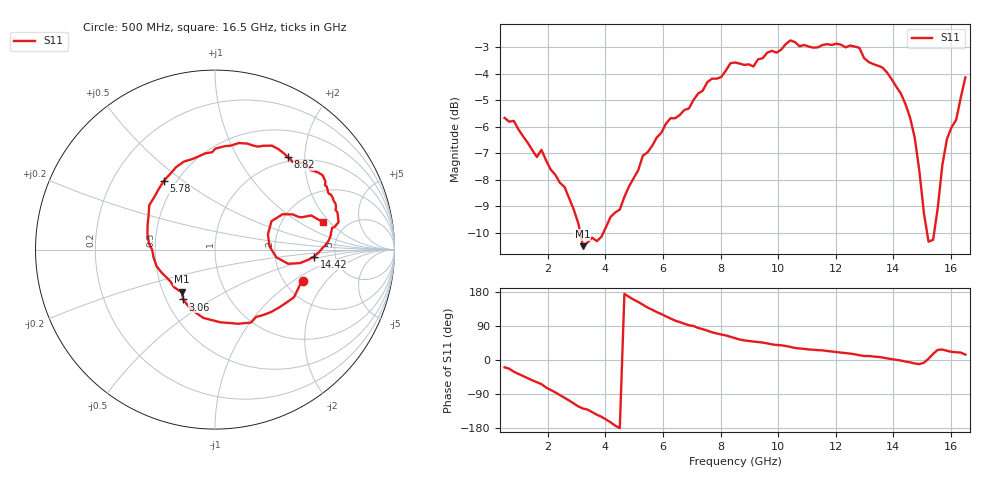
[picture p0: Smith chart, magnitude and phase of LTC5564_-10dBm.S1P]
! LTC5564 S11 -10 dBm source power.
! Reference plane is 1.1 mm from edge of QFN package.
! Measured 11-Jan 2013
# GHZ S DB R 50
!GHz	dB_S11	angS11
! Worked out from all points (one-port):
!   101 points, 500 MHz to 16.5 GHz, reference 50 ohm
!   lowest |S11| = -10.5 dB at 3.22 GHz (marker M1), VSWR 1.85, Z = 31.3 - j16.1 ohm
!   |S11| at or under -10 dB: 3.127 GHz to 3.925 GHz (797.9 MHz wide, 22.6 % of centre); 15.17 GHz to 15.41 GHz (244 MHz wide, 1.6 % of centre)
!   S11 on the Smith chart (normalised r, x): 500 MHz: 2.53, -1.20; 3.06 GHz: 0.61, -0.38; 5.78 GHz: 0.43, +0.43; 8.82 GHz: 0.92, +1.66; 14.42 GHz: 3.42, -0.38; 16.5 GHz: 3.38, +1.68
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0.5  -5.67 -19.4
0.98  -6.10 -36.6
1.78  -6.87 -63.8
2.58  -8.27 -99.7
3.06  -9.64 -122.6
3.22  -10.50 -128.1
4.02  -9.78 -156.9
4.5  -9.12 -179.7
5.3  -7.09 146.0
5.78  -6.41 126.6
6.26  -5.68 109.5
6.58  -5.56 100.1
7.54  -4.32 77.5
8.5  -3.58 57.7
8.82  -3.67 51.8
10.26  -2.89 36.9
10.58  -2.81 31.8
12.5  -2.94 16.9
12.98  -3.41 10.6
13.62  -3.77 6.6
14.42  -5.15 -4.0
14.58  -5.66 -6.3
14.9  -7.65 -10.9
15.22  -10.33 3.3
15.38  -10.26 16.2
15.7  -7.44 27.6
16.34  -4.90 19.5
16.5  -4.14 14.2
